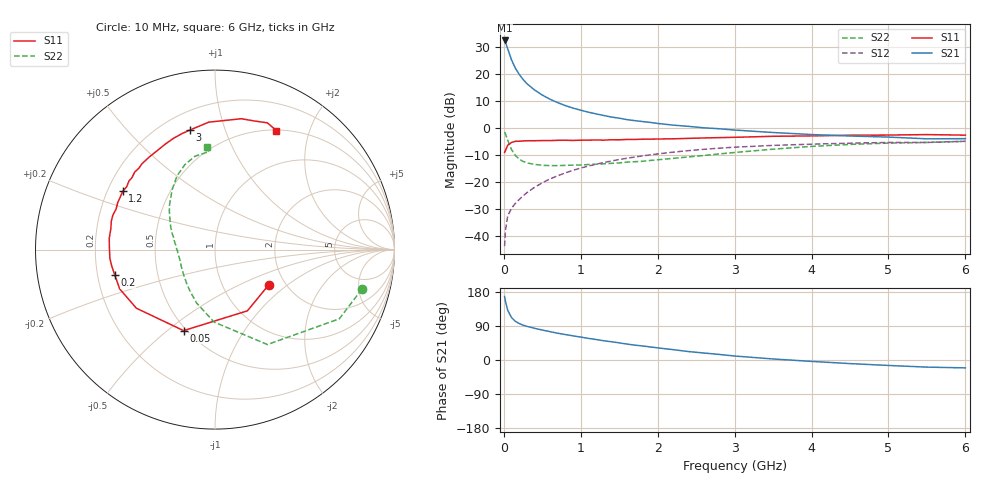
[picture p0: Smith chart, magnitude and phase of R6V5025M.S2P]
! SIEMENS Small Signal Semiconductors
! BFR193
! Si NPN RF Bipolar Junction Transistor in SOT23
! VCE = 0.5 V  IC = 25 mA
! Common Emitter S-Parameters:  May  1996
# GHz  S  MA  R  50
!  f  S11  S21  S12  S22
! GHz  MAG  ANG  MAG  ANG  MAG  ANG  MAG  ANG
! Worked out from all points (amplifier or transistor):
!   36 points, 10 MHz to 6 GHz, reference 50 ohm
!   highest |S21| = 32.5 dB at 10 MHz (marker M1)
!   |S21| within 3 dB of that: start of sweep to 48.88 MHz
!   unconditionally stable (mu >= 1): 355.3 MHz to 3.096 GHz; 3.891 GHz to 4.11 GHz; 5.017 GHz to end of sweep
!   at 250 MHz: K = 0.93, MSG = 21.5 dB, |S12| = -25.0 dB
!   at 1.4 GHz: K = 1.06, MAG = 6.6 dB, |S12| = -12.1 dB
!   at 6 GHz: K = 1.01, MAG = -0.1 dB, |S12| = -4.8 dB
!   S11 on the Smith chart (normalised r, x): 10 MHz: 1.64, -0.74; 50 MHz: 0.48, -0.57; 200 MHz: 0.27, -0.12; 1.2 GHz: 0.26, +0.27; 3 GHz: 0.31, +0.76; 6 GHz: 0.51, +1.52
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0.01  0.358 -33.4  42.09 167.5  0.0066 78.2  0.8482 -15.0
0.02  0.386 -62.1  39.64 155.7  0.0125 70.2  0.7927 -29.1
0.05  0.4843 -111.2  29.47 131.3  0.024 58.4  0.6042 -61.1
0.1  0.5464 -143.3  18.39 112.0  0.0331 54.0  0.4036 -90.8
0.15  0.5744 -157.6  12.89 102.0  0.0409 56.0  0.314 -109.2
0.2  0.5759 -165.6  9.938 96.3  0.0482 58.9  0.2687 -121.4
0.25  0.5829 -171.1  8.003 92.0  0.0561 60.7  0.2438 -130.8
0.3  0.5878 -175.3  6.69 88.8  0.0644 63.1  0.229 -137.9
0.4  0.5888 178.3  5.099 83.6  0.0811 64.6  0.2145 -149.1
0.5  0.5926 173.7  4.114 79.1  0.0982 65.5  0.2069 -157.0
0.6  0.5918 168.8  3.445 74.8  0.1154 65.3  0.2039 -162.6
0.7  0.5991 164.6  2.979 70.7  0.1324 64.7  0.204 -167.3
0.9  0.5955 157.6  2.36 63.7  0.1672 62.8  0.2079 -175.6
1.1  0.6036 151.1  1.986 57.1  0.2001 60.1  0.2137 179.1
1.2  0.6078 147.6  1.844 54.0  0.2169 58.6  0.217 176.1
1.6  0.6218 136.0  1.446 42.1  0.279 52.0  0.2365 166.3
2.2  0.6388 120.1  1.144 27.3  0.3622 41.6  0.2775 152.8
3  0.6804 102.0  0.927 10.5  0.447 27.6  0.3566 135.2
3.5  0.711 92.8  0.835 2.7  0.4822 19.4  0.4107 125.5
4.5  0.7439 78.6  0.72 -9.5  0.5306 5.9  0.5029 109.4
5.5  0.7642 67.6  0.638 -18.8  0.5473 -6.5  0.5466 93.5
6  0.7465 62.7  0.643 -20.8  0.5751 -10.3  0.5733 94.5
